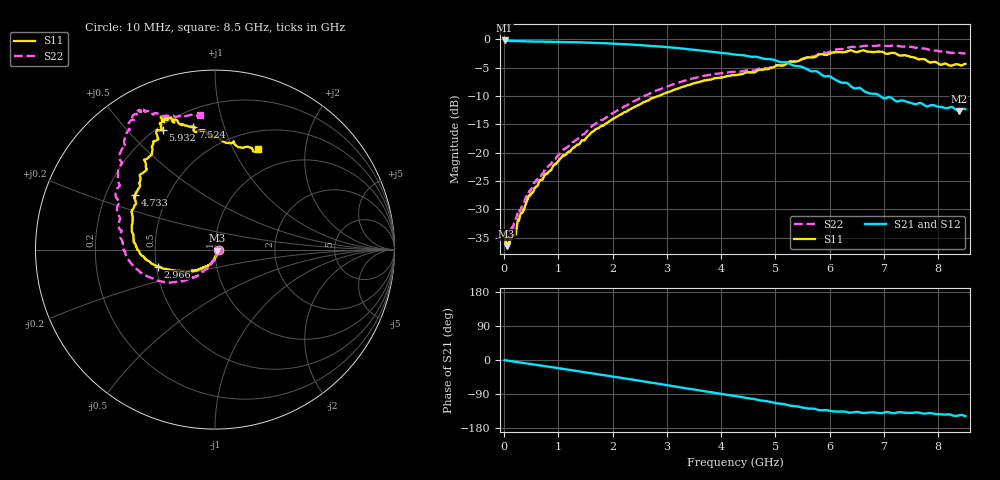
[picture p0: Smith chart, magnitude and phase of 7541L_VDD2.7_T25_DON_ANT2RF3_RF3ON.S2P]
!Agilent Technologies,E5071C,MY46417908,A.11.23
!Date: Wed Dec 09 17:18:04 2020
!Data & Calibration Information:
!Freq	S11:SOLT2(ON)	S21:SOLT2(ON)	S12:SOLT2(ON)	S22:SOLT2(ON)
!PortZ  Port1:50+j0  Port2:50+j0
!Above PortZ is port z conversion or system Z0 setting when saving the data.
!When reading, reference impedance value at option line is always used.
# Hz S dB R 50
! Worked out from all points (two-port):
!   1601 points, 10 MHz to 8.5 GHz, reference 50 ohm
!   highest |S21| = -0.20 dB at 10 MHz (marker M1); lowest = -12.6 dB at 8.378 GHz (marker M2)
!   |S21| within 3 dB of the highest: start of sweep to 4.696 GHz
!   lowest |S11| = -36.5 dB at 47.14 MHz (marker M3), VSWR 1.03, Z = 51.4 - j0.682 ohm
!   |S11| at or under -10 dB: start of sweep to 2.844 GHz
!   |S22| runs from -35.9 to -1.0 dB; largest |S21 - S12| = 0.0035
!   S11 on the Smith chart (normalised r, x): 10 MHz: 1.04, -0.00; 2.966 GHz: 0.51, -0.11; 4.733 GHz: 0.32, +0.28; 5.932 GHz: 0.22, +0.63; 7.524 GHz: 0.30, +0.79; 8.5 GHz: 0.71, +1.25
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1e7  -34.00 -3.2  -0.20 -0.5  -0.20 -0.5  -35.16 -14.4
4.714375e7  -36.52 -26.4  -0.27 -1.3  -0.27 -1.3  -35.57 -27.9
1.798e8  -34.61 -57.5  -0.31 -4.1  -0.31 -4.1  -32.51 -57.1
4.291938e8  -28.40 -84.3  -0.36 -9.5  -0.37 -9.4  -27.50 -84.9
5.724625e8  -26.15 -91.2  -0.38 -12.4  -0.38 -12.4  -25.18 -93.6
1.060638e9  -20.82 -111.1  -0.46 -22.8  -0.46 -22.8  -19.82 -109.7
1.426769e9  -17.94 -125.0  -0.55 -30.8  -0.55 -30.8  -16.97 -119.2
2.1325e9  -13.34 -145.6  -0.82 -46.5  -0.82 -46.5  -12.30 -134.6
2.843538e9  -10.00 -161.6  -1.25 -62.8  -1.26 -62.8  -8.91 -150.9
2.965581e9  -9.53 -163.6  -1.34 -65.6  -1.34 -65.6  -8.49 -154.0
3.554575e9  -7.60 -176.4  -1.90 -79.3  -1.89 -79.3  -6.72 -168.0
4.255e9  -6.33 162.8  -2.68 -95.1  -2.68 -95.0  -5.75 176.5
4.732562e9  -5.34 145.7  -3.29 -106.9  -3.28 -106.9  -5.11 165.3
5.236656e9  -4.06 128.4  -4.19 -119.7  -4.18 -119.7  -4.08 152.0
5.671769e9  -3.21 117.2  -5.66 -128.2  -5.62 -128.2  -3.01 137.2
5.931775e9  -2.76 113.7  -6.54 -132.0  -6.52 -132.0  -2.38 130.9
6.425256e9  -2.06 111.9  -8.54 -138.4  -8.56 -138.1  -1.32 122.8
7.088538e9  -2.50 108.3  -10.17 -137.9  -10.19 -138.2  -1.18 118.5
7.52365e9  -3.15 100.4  -11.33 -139.6  -11.34 -139.7  -1.36 115.7
7.942844e9  -3.98 89.2  -11.73 -142.4  -11.76 -142.5  -1.97 110.4
8.377956e9  -4.47 69.6  -12.64 -146.0  -12.65 -146.1  -2.37 99.0
8.5e9  -4.33 66.8  -12.31 -148.3  -12.39 -148.2  -2.41 96.5
